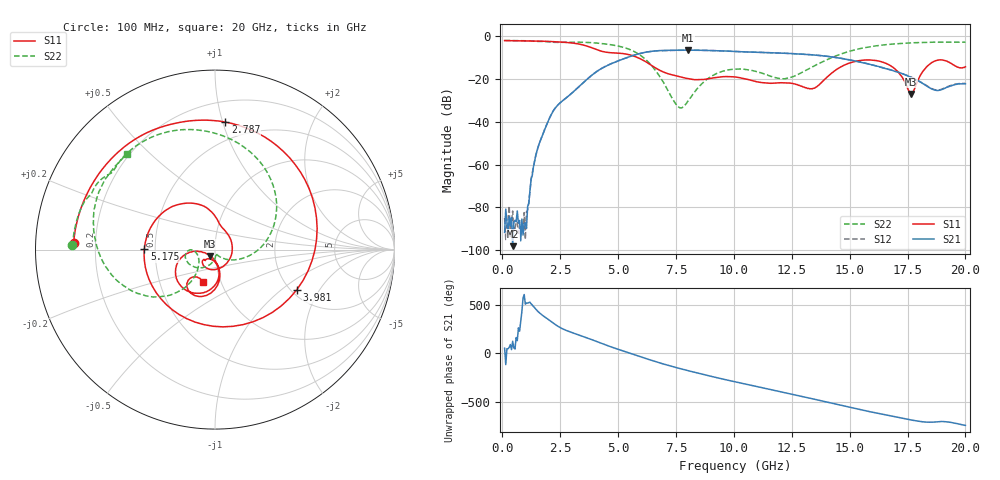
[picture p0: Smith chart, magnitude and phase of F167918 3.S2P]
!  2-Port S-parameters saved by WinCal
! VAR MeasName=S-Parameters (CALIBRATED_DATA) read from VNA (N5242A)
! VAR MeasDate=2016-11-22 10:25:00
! VAR NAME=F167918 3
! VAR FILENAME=F167918 3.S2P
! VAR DATE=2016-11-22 10:25:00
! VAR PHYS_PORTS=1,2
# Hz S DB R 50
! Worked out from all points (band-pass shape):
!   401 points, 100 MHz to 20 GHz, reference 50 ohm
!   highest |S21| = -6.53 dB at 8.01 GHz (marker M1); lowest = -98.2 dB at 448.2 MHz (marker M2)
!   |S21| within 3 dB of the highest: 5.509 GHz to 14.12 GHz (8.607 GHz wide, 87.7 % of centre)
!   lowest |S11| = -27.1 dB at 17.66 GHz (marker M3), VSWR 1.09, Z = 47.3 - j3.41 ohm
!   |S11| at or under -10 dB: 5.842 GHz to end of sweep
!   |S22| runs from -33.5 to -2.0 dB; largest |S21 - S12| = 0.0034
!   S11 on the Smith chart (normalised r, x): 100 MHz: 0.12, +0.02; 2.787 GHz: 0.35, +1.02; 3.981 GHz: 2.14, -1.29; 5.175 GHz: 0.43, +0.00; 20 GHz: 0.82, -0.31
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1e8  -2.07 177.3  -91.72 53.5  -85.04 12.4  -2.00 178.3
4.4825e8  -2.11 168.0  -98.15 124.5  -81.72 -69.9  -2.04 172.5
1.04525e9  -2.21 151.8  -89.84 156.1  -82.10 152.7  -2.15 162.4
1.64225e9  -2.33 133.7  -48.88 45.9  -48.80 46.2  -2.43 153.2
2.7865e9  -2.94 85.3  -28.61 -127.3  -28.62 -127.7  -2.79 135.7
3.43325e9  -3.96 37.6  -22.36 178.4  -22.39 178.3  -2.83 121.7
3.9805e9  -5.89 -26.2  -17.29 130.5  -17.28 130.6  -3.13 107.3
4.478e9  -7.48 -98.5  -14.02 85.6  -13.96 85.5  -3.68 92.1
5.1745e9  -8.09 179.6  -10.84 28.9  -10.81 28.4  -5.06 65.2
5.9705e9  -10.63 118.2  -8.01 -33.3  -8.05 -33.7  -8.98 22.5
6.7665e9  -15.75 84.6  -6.76 -94.3  -6.79 -94.4  -18.32 -28.4
7.5625e9  -18.73 57.5  -6.55 -147.5  -6.58 -147.5  -32.64 -73.6
8.01025e9  -19.83 27.3  -6.53 -175.0  -6.55 -175.0  -30.47 -79.1
8.90575e9  -19.90 -54.1  -6.66 132.7  -6.65 132.7  -19.58 -116.2
1.005e10  -19.07 -121.9  -7.12 70.3  -7.13 70.4  -15.40 -158.6
1.159225e10  -22.03 -133.9  -7.73 -8.5  -7.73 -8.6  -18.77 -176.7
1.338325e10  -24.60 -106.2  -8.71 -102.4  -8.70 -102.2  -14.40 -127.1
1.507475e10  -12.27 -103.3  -11.25 166.8  -11.20 166.8  -6.82 -145.4
1.67165e10  -13.51 -163.0  -15.57 84.6  -15.59 84.7  -3.83 -177.7
1.766175e10  -27.06 -126.0  -19.22 40.1  -19.12 40.7  -3.12 166.1
1.865675e10  -11.71 -100.5  -25.10 19.2  -24.98 19.5  -2.80 150.2
2e10  -14.31 -110.6  -22.24 -15.5  -22.07 -15.5  -2.80 132.6
